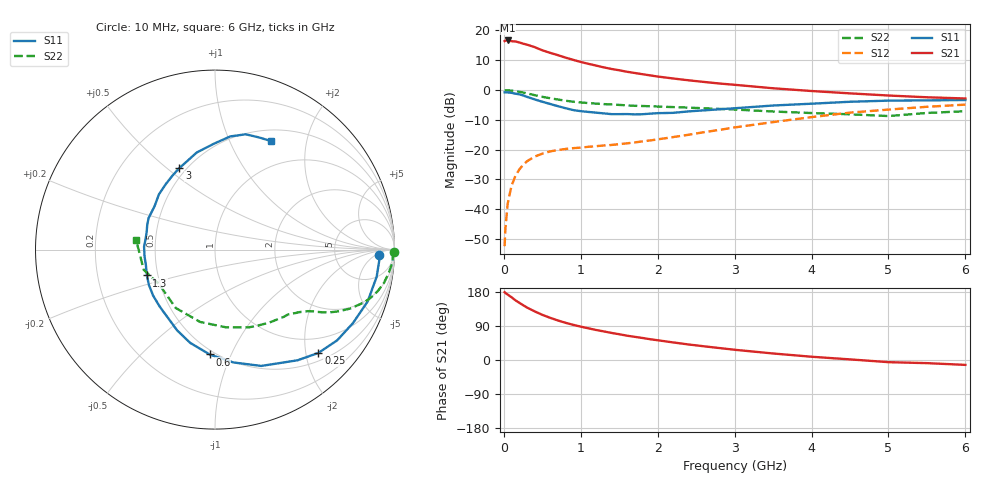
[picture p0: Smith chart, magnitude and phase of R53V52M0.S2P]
! SIEMENS Small Signal Semiconductors
! BFR183
! Si NPN RF Bipolar Junction Transistor in SOT23
! VCE = 3.5 V  IC = 2 mA
! Common Emitter S-Parameters:  May  1996
# GHz  S  MA  R  50
!  f  S11  S21  S12  S22
! GHz  MAG  ANG  MAG  ANG  MAG  ANG  MAG  ANG
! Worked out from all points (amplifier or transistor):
!   36 points, 10 MHz to 6 GHz, reference 50 ohm
!   highest |S21| = 16.7 dB at 50 MHz (marker M1)
!   |S21| within 3 dB of that: start of sweep to 471.4 MHz
!   unconditionally stable (mu >= 1): 1.389 GHz to 2.837 GHz
!   at 250 MHz: K = 0.23, MSG = 20.3 dB, |S12| = -25.1 dB
!   at 1.4 GHz: K = 1.01, MAG = 12.3 dB, |S12| = -18.4 dB
!   at 6 GHz: K = 0.91, MSG = 1.0 dB, |S12| = -4.9 dB
!   S11 on the Smith chart (normalised r, x): 10 MHz: 20, -8; 250 MHz: 0.66, -2.25; 600 MHz: 0.47, -0.83; 1.3 GHz: 0.43, -0.15; 3 GHz: 0.46, +0.55; 6 GHz: 0.64, +1.44
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0.01  0.9167 -1.9  6.636 178.9  0.0024 89.1  0.9962 -0.8
0.02  0.917 -3.9  6.743 176.9  0.0047 86.8  0.991 -1.5
0.05  0.9134 -9.5  6.801 172.6  0.0124 84.7  0.9921 -3.9
0.1  0.8983 -18.8  6.61 165.6  0.0248 80.9  0.9772 -7.5
0.15  0.8708 -28.1  6.535 157.6  0.0361 74.1  0.9599 -11.1
0.2  0.8478 -36.6  6.308 151.1  0.0463 69.5  0.9359 -14.3
0.25  0.8143 -45.0  6.004 144.8  0.0555 65.3  0.9089 -17.1
0.3  0.7692 -53.3  5.788 138.5  0.0637 62.0  0.8814 -19.5
0.4  0.6976 -68.3  5.258 128.4  0.0764 55.6  0.8213 -23.6
0.5  0.6368 -80.8  4.648 119.2  0.0856 50.8  0.7698 -26.5
0.6  0.585 -92.9  4.223 111.5  0.0934 47.4  0.7306 -28.6
0.8  0.497 -115.1  3.51 98.3  0.1026 43.4  0.6634 -31.5
0.9  0.4621 -124.5  3.218 92.9  0.1059 42.9  0.6377 -32.6
1.1  0.4294 -143.5  2.757 83.6  0.1117 42.7  0.605 -34.9
1.3  0.406 -159.2  2.401 75.4  0.1174 43.4  0.5814 -36.9
1.6  0.3955 177.7  2.03 64.2  0.1276 46.4  0.5541 -40.4
2.2  0.4145 144.4  1.565 46.4  0.1626 52.9  0.518 -49.3
3  0.4952 113.7  1.226 27.0  0.236 53.9  0.4715 -66.9
3.5  0.5507 100.6  1.072 17.2  0.2901 50.5  0.4367 -82.2
4.5  0.6364 82.3  0.88 1.6  0.4179 38.9  0.3919 -123.9
5.5  0.6714 68.5  0.757 -8.3  0.524 24.2  0.4129 -164.2
6  0.6804 62.7  0.722 -12.9  0.5696 15.0  0.4416 173.4
